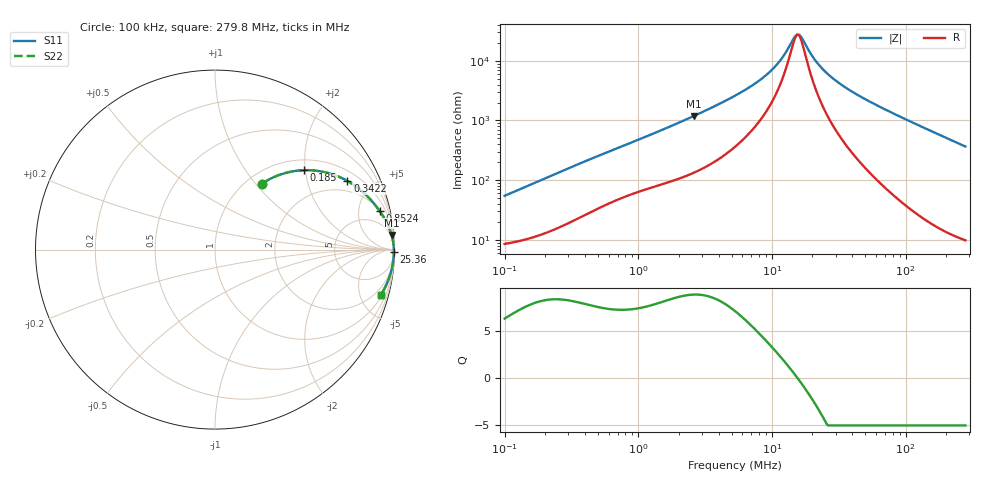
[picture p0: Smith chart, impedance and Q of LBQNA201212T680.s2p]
! LBQNA201212T680  S-PARAMETER MODEL  ( General Type )
! Model Generated by TAIYO YUDEN Corporation (http://www.ty-top.com)
! Version 1.0
! TAIYO YUDEN Control No. 191025NI43SB-FBB
! Copyright(c) 2019 TAIYO YUDEN CO.,LTD. All Rights Reserved.
! Product Description (link to TY-COMPAS)
! https://ds.yuden.co.jp/TYCOMPAS/or/detail?pn=LBQNA201212T680K&u=M
! Products Name : Inductors
! Characteristics :
!  Inductance : 68 uH , SRF(min) : 10 MHz , DC Resistance(max) : 7.8 Ohm
!  Rated Current : Saturation :70 mA , Temp Rise : 100 mA (20 degC)
!  Case Size : 2.0 x 1.25 / 0.079 x 0.049 [mm/inch] , Thickness : 1.25 / 0.049 [mm/inch]
!  (Conditions: Temperature = 25 degC , DC Bias Current/Voltage = 0A / 0V)
! External Node Assignments :
!  1  o---GGG---o  2
! GND o---------o GND
! Frequency Range : 0.1MHz  -  279.750408MHz  [ 402 STEP ]
# MHz S RI R 50
! Freq[MHz].  S11 Real  S11 Imag  S21 Real  S21 Imag  S12 Real  S12 Imag  S22 Real  S22 Imag
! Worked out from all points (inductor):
!   401 points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, 100 kHz to 279.8 MHz, reference 50 ohm
!   read as one part in series: L = 85.5 uH near 104 kHz
!   highest Q = 8.86 at 2.589 MHz (marker M1), where L = 72.2 uH
!   self-resonance near 15.44 MHz
!   S11 on the Smith chart (normalised r, x): 100 kHz: 1.17, +1.08; 185 kHz: 1.24, +1.97; 342.2 kHz: 1.44, +3.55; 852.4 kHz: 2.12, +8.15; 25.36 MHz: open; 279.8 MHz: 1.20, -7.32
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0.1  0.2614 0.3673  0.7386 -0.3673  0.7386 -0.3673  0.2614 0.3673
0.18498  0.4968 0.4425  0.5032 -0.4425  0.5032 -0.4425  0.4968 0.4425
0.342176  0.7372 0.3827  0.2628 -0.3827  0.2628 -0.3827  0.7372 0.3827
0.377863  0.7671 0.3645  0.2329 -0.3645  0.2329 -0.3645  0.7671 0.3645
0.550878  0.8551 0.2911  0.1449 -0.2911  0.1449 -0.2911  0.8551 0.2911
0.85237  0.9181 0.214  0.0819 -0.214  0.0819 -0.214  0.9181 0.214
1.427803  0.9606 0.1416  0.0394 -0.1416  0.0394 -0.1416  0.9606 0.1416
2.589262  0.9838 0.0819  0.0162 -0.0819  0.0162 -0.0819  0.9838 0.0819
5.289144  0.9932 0.0376  0.00675 -0.0376  0.00675 -0.0376  0.9932 0.0376
7.559447  0.995 0.023  0.00504 -0.023  0.00504 -0.023  0.995 0.023
9.979919  0.9957 0.0135  0.00428 -0.0135  0.00428 -0.0135  0.9957 0.0135
11.69668  0.996 0.00856  0.00397 -0.00856  0.00397 -0.00856  0.996 0.00856
14.54952  0.9963 0.00202  0.00367 -0.00202  0.00367 -0.00202  0.9963 0.00202
15.44185  0.9964 0.000255  0.00361 -0.000255  0.00361 -0.000255  0.9964 0.000255
16.06694  0.9964 -0.000923  0.00358 0.000923  0.00358 0.000923  0.9964 -0.000923
16.71734  0.9965 -0.00211  0.00355 0.00211  0.00355 0.00211  0.9965 -0.00211
19.9857  0.9965 -0.00752  0.00346 0.00752  0.00346 0.00752  0.9965 -0.00752
25.35844  0.9965 -0.0152  0.00348 0.0152  0.00348 0.0152  0.9965 -0.0152
38.46609  0.9959 -0.0311  0.00407 0.0311  0.00407 0.0311  0.9959 -0.0311
75.51853  0.9919 -0.0699  0.00813 0.0699  0.00813 0.0699  0.9919 -0.0699
148.2617  0.9759 -0.1396  0.0241 0.1396  0.0241 0.1396  0.9759 -0.1396
279.7504  0.9247 -0.2508  0.0753 0.2508  0.0753 0.2508  0.9247 -0.2508
